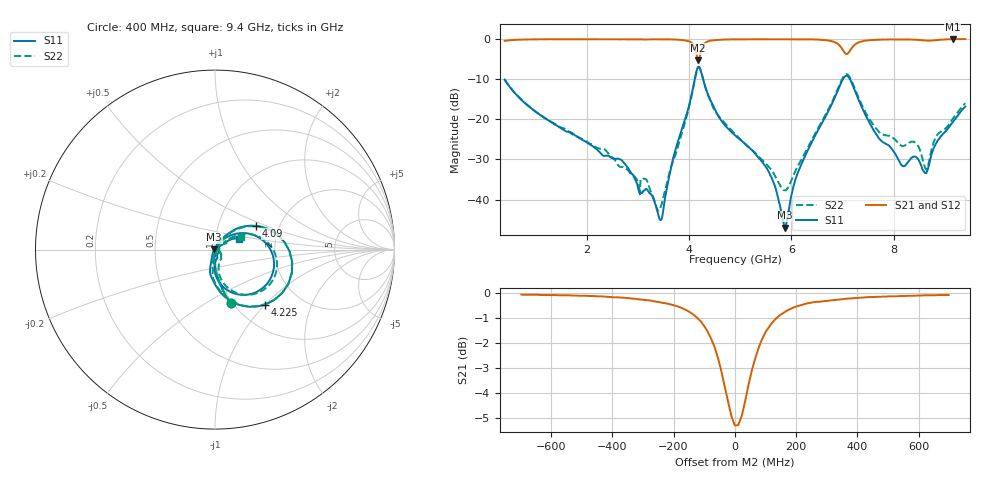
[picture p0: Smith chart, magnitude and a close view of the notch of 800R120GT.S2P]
!  American Technical Ceramics  Date:  10/25/10
!  One Norden Lane
!  Huntington Station,  NY.  11746-2102
!  Tel:  (631) 622-4700  Fax:  (631) 622-4748
!  Part Number  800R120GT.TXT  Mounting Orientation: Horizontal
!  Description: Ultra Low ESR Microwave Capacitor
!  Application: Coupling, Bypass, Tuning, DC Block, Filters, Matching
# GHZ S DB R 50
! Freq  |S11|  S11 Ph  |S21|  S21 Ph  |S12|  S12 Ph  |S22|  S22 Ph
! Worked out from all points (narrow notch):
!   801 points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, 400 MHz to 9.4 GHz, reference 50 ohm
!   highest |S21| = -0.01 dB at 9.153 GHz (marker M1); lowest = -5.3 dB at 4.18 GHz (marker M2)
!   notch at M2: 5.2 dB deep, 118 MHz wide at half that depth
!   lowest |S11| = -47.0 dB at 5.879 GHz (marker M3), VSWR 1.01, Z = 49.6 + j0.169 ohm
!   |S11| at or under -10 dB: start of sweep to 4.115 GHz; 4.277 GHz to 7.008 GHz (2.731 GHz wide, 48.4 % of centre); 7.145 GHz to end of sweep
!   |S22| runs from -42.8 to -6.9 dB; largest |S21 - S12| = 0.0013
!   S11 on the Smith chart (normalised r, x): 400 MHz: 0.98, -0.65; 4.09 GHz: 1.52, +0.43; 4.225 GHz: 1.35, -1.00; 9.4 GHz: 1.29, +0.15
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0.4  -10.12 -73.5  -0.45 16.4  -0.45 16.4  -10.09 -73.6
1.908  -25.05 -94.4  -0.04 -5.4  -0.04 -5.4  -24.90 -95.1
2.718  -30.67 -91.6  -0.07 -10.7  -0.07 -10.7  -31.89 -93.1
3.156  -37.38 -59.5  -0.12 -13.6  -0.12 -13.6  -34.95 -70.3
3.404  -43.93 -29.1  -0.06 -15.4  -0.06 -15.4  -42.74 -23.8
4.09  -11.53 29.9  -1.51 -31.9  -1.51 -31.9  -11.80 30.5
4.18  -6.97 -17.3  -5.28 -20.3  -5.28 -20.3  -7.01 -16.3
4.225  -7.65 -47.6  -3.64 -1.5  -3.64 -1.5  -7.64 -47.0
4.371  -13.81 -88.3  -0.58 -7.9  -0.58 -7.9  -13.90 -87.4
4.9  -24.00 -108.2  -0.08 -17.7  -0.08 -17.7  -23.64 -101.0
5.53  -32.44 -121.1  -0.06 -22.5  -0.06 -22.5  -31.45 -84.0
5.879  -47.01 157.6  -0.05 -24.9  -0.05 -24.9  -37.69 -29.0
6.408  -25.47 56.1  -0.09 -29.7  -0.09 -29.6  -24.93 38.2
6.903  -12.97 21.9  -1.16 -39.6  -1.16 -39.6  -12.60 20.2
7.083  -9.15 -29.6  -3.74 -28.7  -3.74 -28.7  -8.77 -27.3
7.319  -15.28 -84.4  -0.81 -20.2  -0.81 -20.2  -14.76 -76.9
7.904  -26.52 -73.5  -0.11 -29.4  -0.11 -29.4  -24.09 -54.7
8.174  -31.68 -49.3  -0.10 -31.7  -0.10 -31.7  -26.70 -38.8
8.433  -29.39 -26.3  -0.18 -33.8  -0.18 -33.8  -25.90 -32.4
8.635  -33.43 8.7  -0.39 -34.4  -0.39 -34.4  -32.56 -0.9
9.153  -20.73 33.8  -0.01 -35.0  -0.01 -35.1  -19.87 35.4
9.4  -16.85 23.9  -0.01 -37.4  -0.01 -37.4  -15.98 25.2
